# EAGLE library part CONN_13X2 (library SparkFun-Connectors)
Multi connection point. Often used as Generic Header-pin footprint for 0.1 inch spaced/style header connections On any of the 0.1 inch spaced packages, you can populate with these: Break Away Headers - Straight (PRT-00116) Break Away Male Headers - Right Angle (PRT-00553) Female Headers (PRT-00115) Break Away Headers - Machine Pin (PRT-00117) Break Away Female Headers - Swiss Machine Pin (PRT-00743)
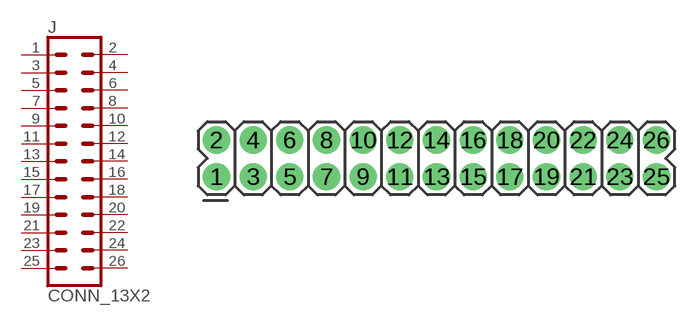
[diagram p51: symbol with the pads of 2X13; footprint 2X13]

Designator prefix J

## CONN_13X22X13  [2X13]
1  1  pas
2  2  pas
3  3  pas
4  4  pas
5  5  pas
6  6  pas
7  7  pas
8  8  pas
9  9  pas
10  10  pas
11  11  pas
12  12  pas
13  13  pas
14  14  pas
15  15  pas
16  16  pas
17  17  pas
18  18  pas
19  19  pas
20  20  pas
21  21  pas
22  22  pas
23  23  pas
24  24  pas
25  25  pas
26  26  pas

## Footprint 2X13 (pad centres in mm)
Plated Through Hole - 2x13 Specifications: Pin count:26 Pin pitch:0.1" Example device(s): CONN_13x2
drill 1.016 pad 1.88: 1 0,0; 2 0,2.54; 3 2.54,0; 4 2.54,2.54; 5 5.08,0; 6 5.08,2.54; 7 7.62,0; 8 7.62,2.54; 9 10.16,0; 10 10.16,2.54; 11 12.7,0; 12 12.7,2.54; 13 15.24,0; 14 15.24,2.54; 15 17.78,0; 16 17.78,2.54; 17 20.32,0; 18 20.32,2.54; 19 22.86,0; 20 22.86,2.54; 21 25.4,0; 22 25.4,2.54; 23 27.94,0; 24 27.94,2.54; 25 30.48,0; 26 30.48,2.54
